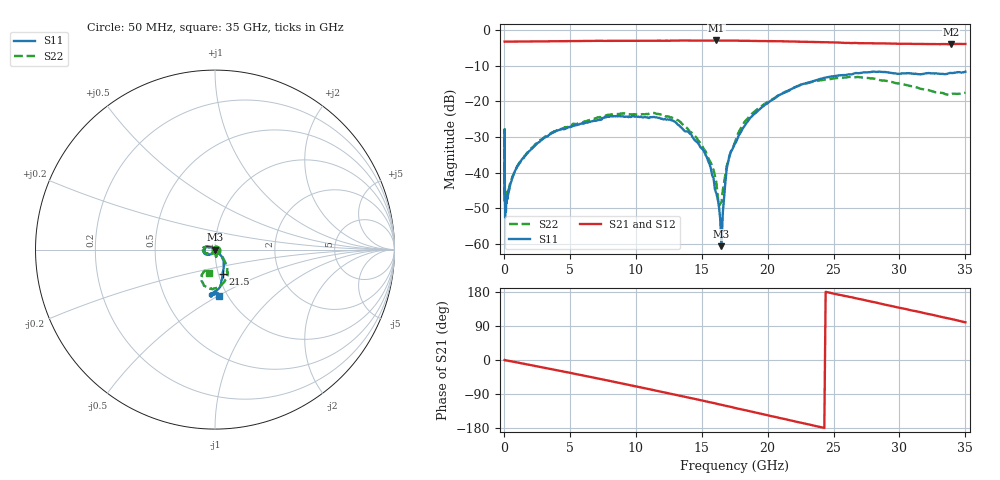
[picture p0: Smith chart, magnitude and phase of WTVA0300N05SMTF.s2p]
! 50 ohm 2-Port S-parameters measured by Modelithics Inc support@modelithics.com  Tampa, FL USA 813-866-6335 (February 2024)
! Smiths Interconnect,  3dB P/N: WTVA0300N05SMTF, Temperature: 25C
! Board: 10 mil Rogers 4350B, Mounting Pad Dimensions: Length: 15 mils, Width: 25 mils, Gap: 40 mils.
# Hz S MA R 50
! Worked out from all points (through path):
!   486 points, 50 MHz to 35 GHz, reference 50 ohm
!   highest |S21| = -2.84 dB at 16.1 GHz (marker M1); lowest = -3.9 dB at 33.9 GHz (marker M2)
!   group delay of S21, straight-line fit = 20.8 ps
!   lowest |S11| = -60.7 dB at 16.5 GHz (marker M3), VSWR 1.00, Z = 50 - j0.0841 ohm
!   |S11| at or under -10 dB: start of sweep to end of sweep
!   |S22| runs from -49.8 to -13.1 dB; largest |S21 - S12| = 0.015
!   S11 on the Smith chart (normalised r, x): 50 MHz: 1.01, -0.00; 21.5 GHz: 1.05, -0.29; 35 GHz: 0.91, -0.51
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5e7  0.005246 -27.3  0.6937 -0.4  0.6935 -0.3  0.004592 -10.9
8e7  0.004833 -41.4  0.6944 -0.5  0.6934 -0.5  0.004939 -11.9
9e7  0.002332 -47.0  0.6941 -0.5  0.6938 -0.5  0.003231 -29.1
1.1e8  0.003328 -37.5  0.6941 -0.7  0.6939 -0.7  0.004157 -32.7
7.5e8  0.009531 -96.8  0.695 -4.9  0.6948 -4.9  0.009706 -92.6
1.8e9  0.01903 -115.9  0.6971 -11.8  0.6969 -11.8  0.01932 -115.8
5.9e9  0.04908 -146.4  0.7082 -40.0  0.7081 -40.1  0.0505 -156.2
1.17e10  0.05868 172.6  0.7152 -82.0  0.7148 -81.9  0.06689 172.8
1.33e10  0.0458 161.5  0.7187 -93.7  0.7188 -93.8  0.05295 161.7
1.49e10  0.0227 149.3  0.7169 -105.8  0.7167 -105.9  0.0259 154.9
1.55e10  0.01433 139.4  0.7182 -110.6  0.7178 -110.6  0.01589 149.7
1.61e10  0.005137 155.5  0.7208 -115.3  0.7207 -115.3  0.007443 123.4
1.63e10  0.003443 163.8  0.7176 -116.8  0.7178 -116.9  0.003364 94.6
1.65e10  0.0009211 -114.0  0.7175 -118.4  0.7174 -118.3  0.003804 32.1
1.7e10  0.01399 -40.2  0.7171 -122.0  0.717 -122.0  0.01416 -22.8
1.76e10  0.02677 -46.3  0.7182 -127.3  0.7183 -127.1  0.02925 -29.7
1.88e10  0.06155 -48.6  0.712 -136.4  0.7119 -136.4  0.06693 -46.6
2.15e10  0.1404 -72.3  0.6987 -157.5  0.6983 -157.3  0.1383 -61.2
2.34e10  0.1917 -79.7  0.6889 -172.3  0.6891 -172.1  0.1886 -74.6
2.92e10  0.2547 -96.1  0.6527 143.9  0.6524 144.4  0.1906 -112.8
3.39e10  0.2517 -85.3  0.6378 108.5  0.6429 108.6  0.1253 -109.4
3.5e10  0.2617 -85.3  0.6434 99.4  0.6428 99.6  0.1326 -103.4
